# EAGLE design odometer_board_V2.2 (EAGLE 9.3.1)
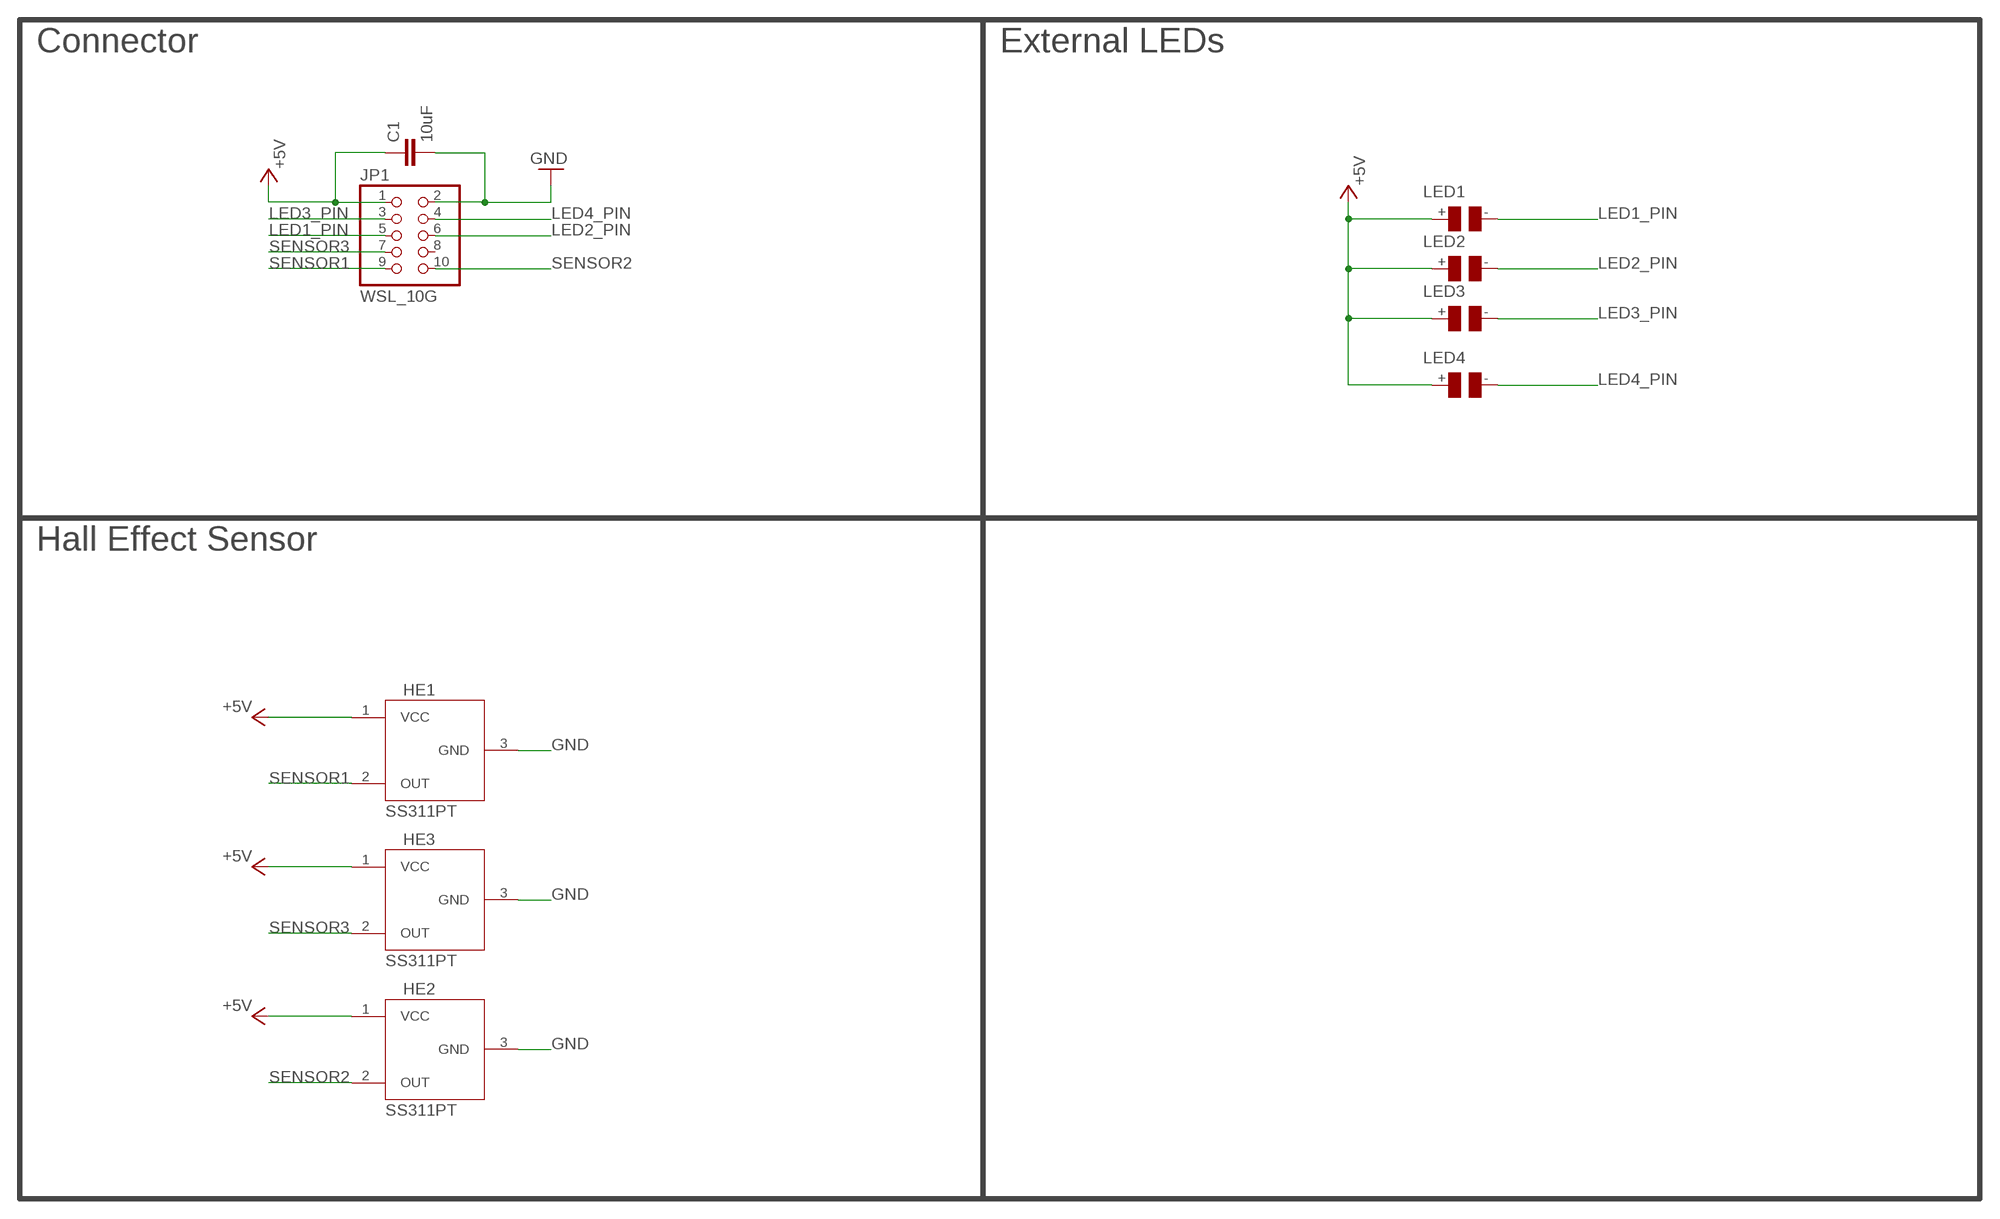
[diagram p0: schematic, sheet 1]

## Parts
C1  10uF  C-EUC0805  [C0805]
HE1  SS311PT  [SOT23]
HE2  SS311PT  [SOT23]
HE3  SS311PT  [SOT23]
JP1  WSL_10G  [WSL_10G]
LED1  EXT_LED  [EXT_LED]
LED2  EXT_LED  [EXT_LED]
LED3  EXT_LED  [EXT_LED]
LED4  EXT_LED  [EXT_LED]

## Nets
+5V: C1.1 HE1.1(VCC) HE2.1(VCC) HE3.1(VCC) JP1.1 LED1.+ LED2.+ LED3.+ LED4.+
GND: C1.2 HE1.3(GND) HE2.3(GND) HE3.3(GND) JP1.2
LED1_PIN: JP1.5 LED1.-
LED2_PIN: JP1.6 LED2.-
LED3_PIN: JP1.3 LED3.-
LED4_PIN: JP1.4 LED4.-
SENSOR1: HE1.2(OUT) JP1.9
SENSOR2: HE2.2(OUT) JP1.10
SENSOR3: HE3.2(OUT) JP1.7
Unconnected: JP1.8

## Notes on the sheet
- Connector | External LEDs
- Hall Effect Sensor

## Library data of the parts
C1 = embedded:C-EU: Capacitor; DESCR: SMD Capacitor; PACKAGE: C0805; SIZE: 0805in
HE1-HE3 = embedded:SS311PT: Hall Effect Sensor; DATASHEET: https://www.mouser.de/datasheet/2/187/ProductSheet_SS311_411-1168392.pdf; DESCR: Digital Switch Latch Open Collector Hall Effect SOT-23-3; DIGIKEY_NO: 480-5345-1-ND; MF: Honeywell; MF_PN: SS311PT; MOUSER_NO: 785-SS311PT; PACKAGE: SOT-23-3; PURCHASE: https://www.mouser.de/ProductDetail/Honeywell/SS311PT?qs=sp0Ey2PL6%252B5pUIwW0wqZZw==; UNIT_PRICE: 1.23000
JP1 = embedded:WSL_10G: Connector WSL 10G WANNENSTECKER, 10-POLIG BOX HEADER Source: Box Header; ANGLE: Straight; DATASHEET: https://cdn-reichelt.de/documents/datenblatt/C151/BH1S-XX-L.pdf; DESCR: Box connector 10pin straight; MF: Amtek; MF_PN: WSL-10G; PACKAGE: Box Header; PITCH: 2.54mm; POS: 10; PURCHASE: https://www.reichelt.de/box-connector-10-pin-straight-wsl-10g-p22816.html?r=1; REICHELT_NO: WSL 10G; ROWS: 2; UNIT_PRICE: 0.1
LED1-LED4 = embedded:EXT_LED: Connector; CONRAD_NO: 405622 - 62; DATASHEET: https://produktinfo.conrad.com/datenblaetter/400000-424999/405622-da-01-en-LED_5MM_NSDW570GS_K1__C0_P10_.pdf; DESCR: LED 5mm Radial; MF: NICHIA; MF_PN: NSDW570GS-K1; PACKAGE: LED 5mm Radial; PURCHASE: https://www.conrad.de/de/p/nichia-nsdw570gs-k1-led-bedrahtet-weiss-rund-5-mm-140-70-ma-3-4-v-405622.html

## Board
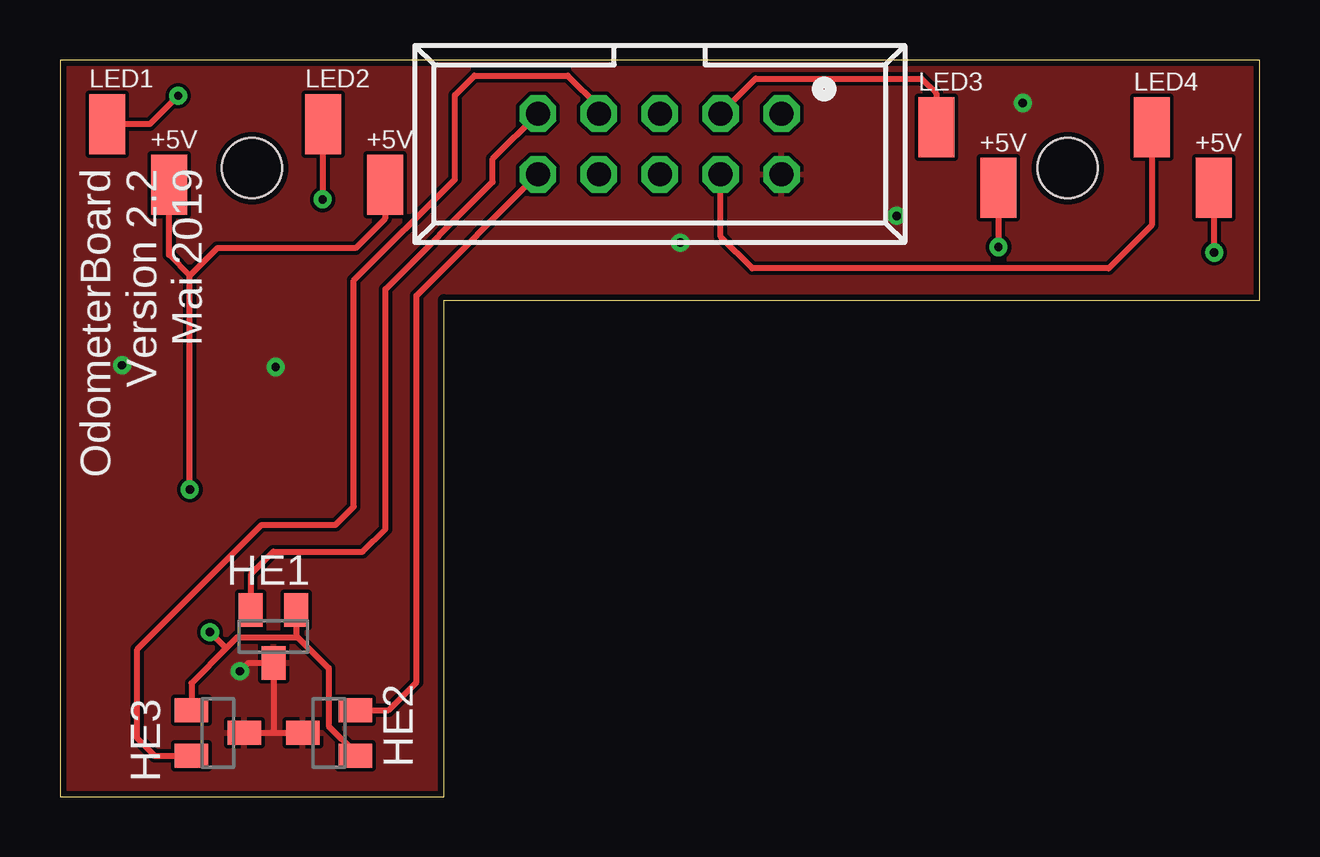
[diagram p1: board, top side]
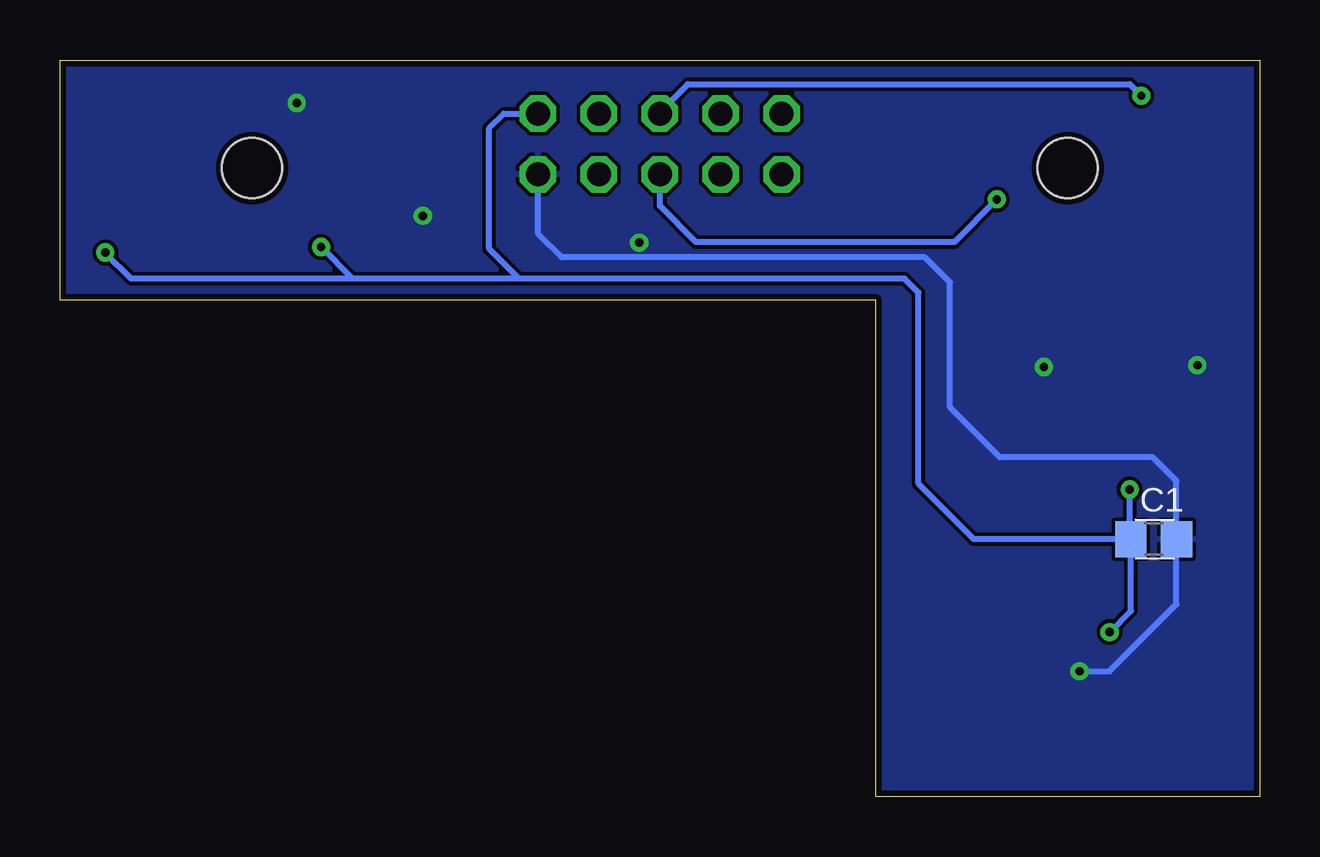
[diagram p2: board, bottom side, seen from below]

Size 50 x 30.7 mm. Coordinates in mm from the lower left corner, seen from the top.
Outline: 0,0 16,0 16,20.7 50,20.7 50,30.7 0,30.7 0,0
Copper layers (1*16): Top 0.035mm / dielectric 1.5mm / Bottom 0.035mm
Design rules "default *": minimum track width 6mil, minimum drill 0.35mm, track to track 6mil, track to pad 6mil, pad to pad 6mil, via to via 6mil, smd to smd 6mil, copper to edge 0.25mm, drill to drill 0.35mm, minimum pad ring 10mil, minimum via ring 8mil, stop-mask expansion 4mil, vias tented up to drill 0mil, thermal gap 6mil
Holes 2.5 mm at 8,26.2 42,26.2

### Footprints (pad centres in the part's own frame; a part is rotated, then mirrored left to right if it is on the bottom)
C0805 = smd 1.3 x 1.5: 1 -0.95,0; 2 0.95,0
SOT23 = smd 1 x 1.4: 1 -0.95,-1.1; 2 0.95,-1.1; 3 0,1.1
WSL_10G = drill 1 octagon: 1 -5.08,-1.27; 2 -5.08,1.27; 3 -2.54,-1.27; 4 -2.54,1.27; 5 0,-1.27; 6 0,1.27; 7 2.54,-1.27; 8 2.54,1.27; 9 5.08,-1.27; 10 5.08,1.27
EXT_LED = smd 1.5 x 2.5: + 1.29,-1.25; - -1.29,1.27

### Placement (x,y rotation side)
C1  4.41,10.74 0 bottom
HE1  8.9,6.68 180 top
HE2  11.22,2.66 90 top
HE3  6.58,2.66 270 top
JP1  25,27.2 180 top
LED1  3.25,26.75 0 top
LED2  12.25,26.75 0 top
LED3  37.82,26.62 0 top
LED4  46.79,26.62 0 top

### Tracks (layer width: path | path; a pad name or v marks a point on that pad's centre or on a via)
+5V  (via drill 0.35)
  Top 0.254: 6.96,6.22 5.48,4.74 HE3.1 | 6.96,6.22 7.39,6.66 9.91,6.66 | 9.91,6.66 11.2,5.36 11.2,2.95 12.32,1.83 HE2.1 | v6.25,6.86 6.89,6.22 6.96,6.22 | HE1.1 9.85,6.71 9.91,6.66 | v48.11,22.68 48.11,25.35 LED4.+ | LED3.+ 39.11,22.92 v39.12,22.91 | LED2.+ 13.54,24.09 12.32,22.86 6.55,22.86 5.41,21.72 | LED1.+ 4.54,22.58 5.41,21.72 | v5.41,12.8 5.41,21.72
  Bottom 0.254: v6.25,6.86 5.36,7.75 C1.1 | 30.86,21.59 14.8,21.59 14.21,21.01 14.21,13.04 11.91,10.74 C1.1 | 30.86,21.59 32.11,22.84 32.11,27.86 31.5,28.47 JP1.1 | 30.86,21.59 37.8,21.59 | 37.8,21.59 47.04,21.59 48.11,22.66 v48.11,22.68 | v39.12,22.91 37.8,21.59 | C1.1 5.41,10.79 v5.41,12.8
GND  (via drill 0.35)
  Top 0.254: v7.5,5.23 7.85,5.58 HE1.3 8.9,2.67 8.89,2.66 | HE3.3 8.89,2.66 | 8.89,2.66 HE2.3
  Bottom 0.254: v7.5,5.23 6.25,5.23 3.46,8.02 C1.2 3.46,13.16 4.45,14.15 10.82,14.15 12.9,16.23 12.9,21.44 13.95,22.48 29.08,22.48 30.07,23.47 JP1.2
  other vias: 8.99,17.91 2.59,17.98 40.13,28.91 25.86,23.09 34.87,24.21
  pour Top: 0.25,30.48 0.25,0.25 15.75,0.25 15.75,20.95 49.78,20.95 49.78,30.48
  pour Bottom: 0.25,30.48 0.25,0.25 15.75,0.25 15.75,20.95 49.78,20.95 49.78,30.48
  pour Bottom: 0.25,30.48 0.25,0.25 15.75,0.25 15.75,20.95 49.78,20.95 49.78,30.48
LED1_PIN  (via drill 0.35)
  Top 0.254: v4.93,29.21 3.74,28.02 LED1.-
  Bottom 0.254: JP1.5 25,28.52 23.83,29.69 5.41,29.69 v4.93,29.21
LED2_PIN  (via drill 0.35)
  Top 0.254: v10.95,24.89 10.96,24.91 LED2.-
  Bottom 0.254: v10.95,24.89 12.72,23.11 23.5,23.11 25,24.62 JP1.6
LED3_PIN
  Top 0.254: JP1.3 28.99,29.92 35.92,29.92 36.53,29.31 LED3.-
LED4_PIN
  Top 0.254: LED4.- 45.5,23.81 43.71,22.02 28.85,22.02 27.54,23.34 JP1.4
SENSOR1
  Top 0.254: HE1.2 7.95,9.27 8.89,10.21 12.62,10.21 13.56,11.15 13.56,21.16 18.03,25.63 18.03,26.58 JP1.9
SENSOR2
  Top 0.254: HE2.2 13.69,3.61 14.86,4.78 14.86,20.88 JP1.10
SENSOR3
  Top 0.254: JP1.7 22.46,28.75 21.16,30.05 17.27,30.05 16.46,29.23 16.46,25.73 12.24,21.51 12.24,12.09 11.48,11.33 8.41,11.33 3.23,6.15 3.23,2.44 3.95,1.71 HE3.2

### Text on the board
tNames: OdometerBoard / Version 2.2 / Mai 2019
